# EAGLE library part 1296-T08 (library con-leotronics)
1.27mm SINGLE ROW FEMALE SOCKET Source: http://www.leotronics.co.uk/Conexcon/Data%20Sheets/sec.%20A/1296ing.pdf
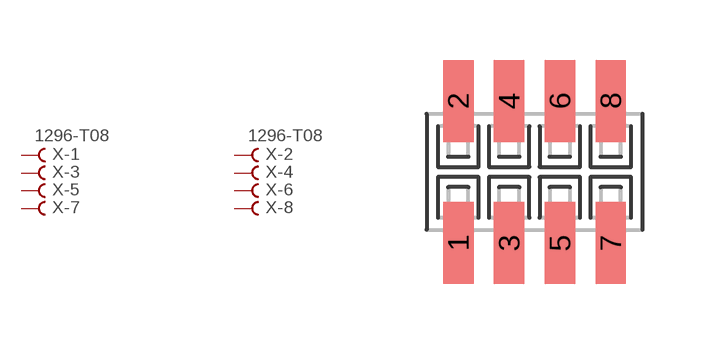
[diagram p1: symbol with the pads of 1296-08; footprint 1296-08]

Designator prefix X; gates -1=FVAL -2=FVAL -3=F -4=F -5=F -6=F -7=F -8=F

## 1296-T08 (OC_FARNELL: unknown; OC_NEWARK: unknown)  [1296-08]
1  -1:B  pas
2  -2:B  pas
3  -3:B  pas
4  -4:B  pas
5  -5:B  pas
6  -6:B  pas
7  -7:B  pas
8  -8:B  pas

## Footprint 1296-08 (pad centres in mm)
1.27mm SINGLE ROW FEMALE SOCKET Source: http://www.leotronics.co.uk/Conexcon/Data%20Sheets/sec.%20A/1296ing.pdf
smd 0.76 x 2.05: 1 -1.905,-1.78; 2 -1.905,1.78; 3 -0.635,-1.78; 4 -0.635,1.78; 5 0.635,-1.78; 6 0.635,1.78; 7 1.905,-1.78; 8 1.905,1.78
